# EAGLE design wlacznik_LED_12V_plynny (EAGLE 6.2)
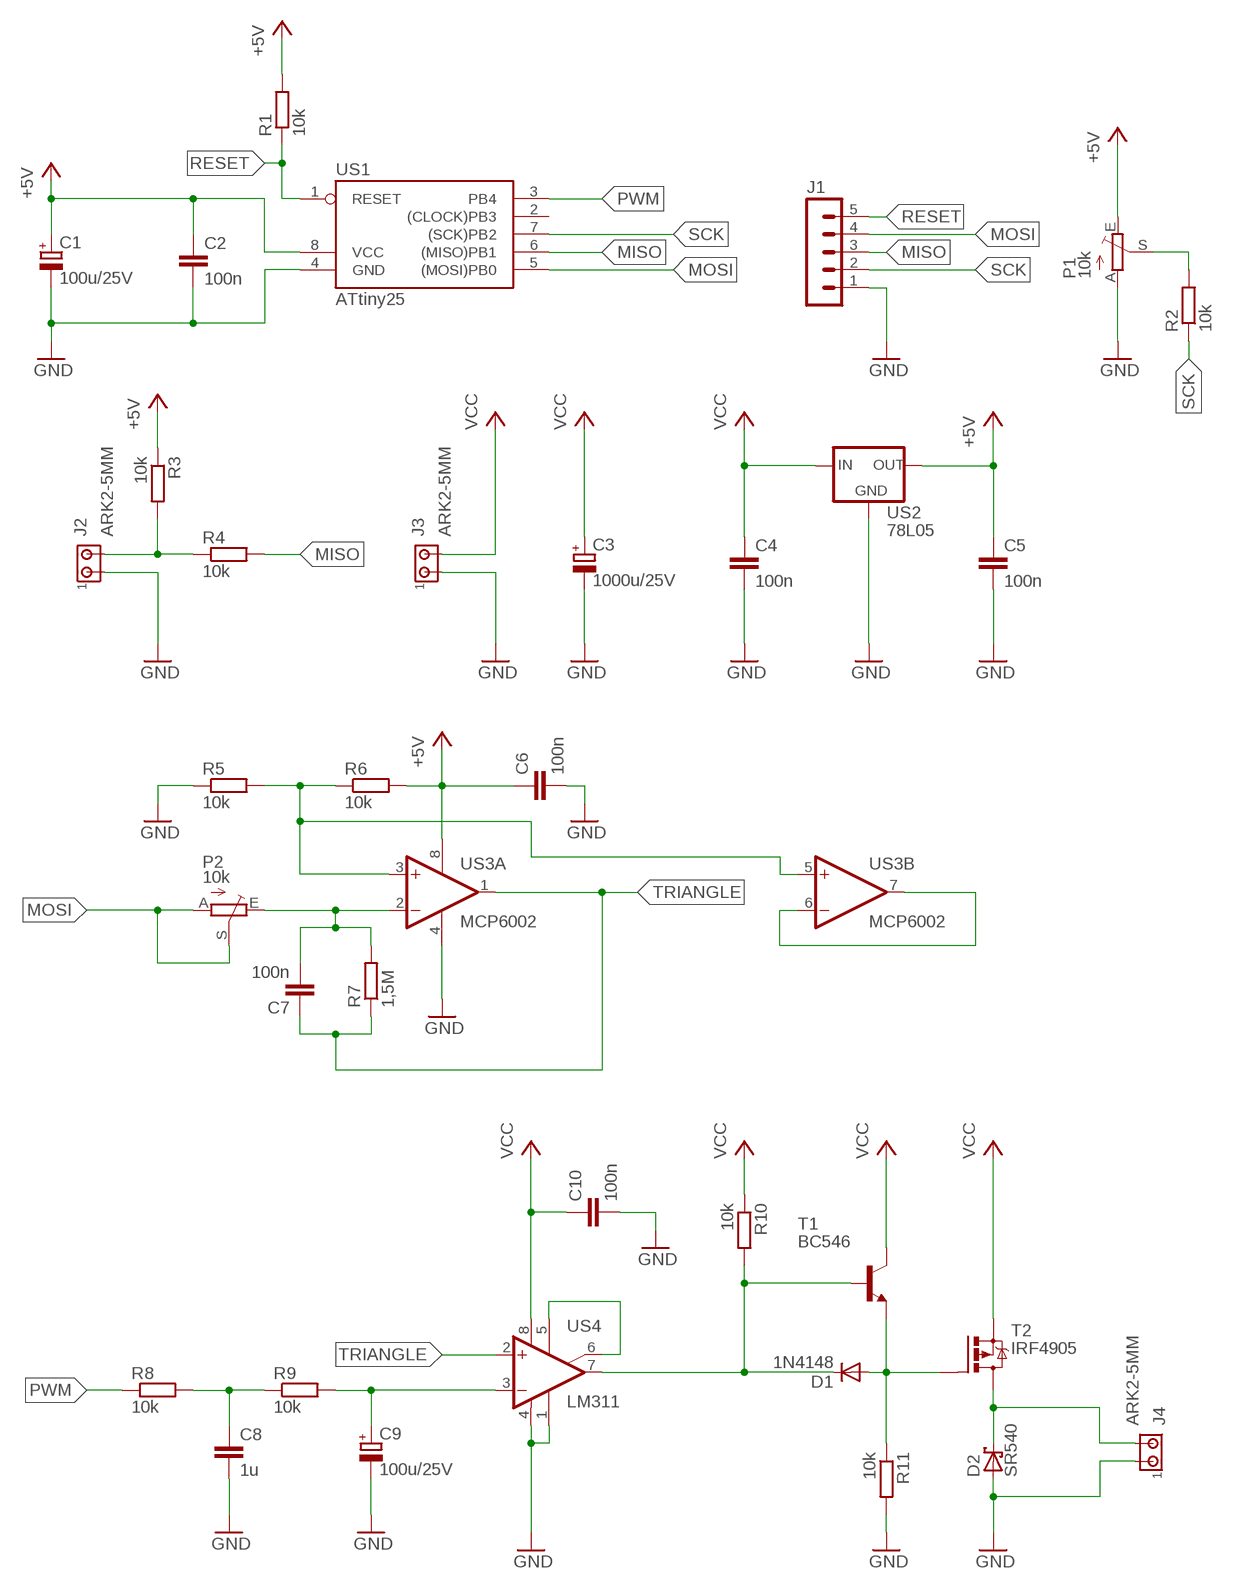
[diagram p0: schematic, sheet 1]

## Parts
C1  100u/25V  CPOL-EUE2.5-6  [E2,5-6]
C2  100n  C-EU050-025X075  [C050-025X075]
C3  1000u/25V  CPOL-EUE5-10.5  [E5-10,5]
C4  100n  C-EU050-025X075  [C050-025X075]
C5  100n  C-EU050-025X075  [C050-025X075]
C6  100n  C-EU050-025X075  [C050-025X075]
C7  100n  C-EU050-025X075  [C050-025X075]
C8  1u  C-EU050-055X075  [C050-055X075]
C9  100u/25V  CPOL-EUE2.5-6  [E2,5-6]
C10  100n  C-EU050-025X075  [C050-025X075]
D1  1N4148  1N4148DO35-7  [DO35-7]
D2  SR540  SCHOTTKY-DIODEC4111-15  [C4111-15]
J1  MA05-1  [MA05-1]
J2  ARK2-5MM  [2PIN-5MM]
J3  ARK2-5MM  [2PIN-5MM]
J4  ARK2-5MM  [2PIN-5MM]
P1  10k  TRIM_EU-CA6V  [CA6V]
P2  10k  TRIM_EU-CA6V  [CA6V]
R1  10k  R-EU_0207/7  [0207/7]
R2  10k  R-EU_0207/7  [0207/7]
R3  10k  R-EU_0207/7  [0207/7]
R4  10k  R-EU_0207/7  [0207/7]
R5  10k  R-EU_0207/7  [0207/7]
R6  10k  R-EU_0207/7  [0207/7]
R7  1,5M  R-EU_0207/7  [0207/7]
R8  10k  R-EU_0207/7  [0207/7]
R9  10k  R-EU_0207/7  [0207/7]
R10  10k  R-EU_0207/7  [0207/7]
R11  10k  R-EU_0207/7  [0207/7]
T1  BC546  BC546A  [TO92-EBC]
T2  IRF4905  IRF9530  [TO220BV]
US1  ATtiny25  TINY22P  [DIL08]
US2  78L05  78LXX  [78LXX]
US3  MCP6002  MCP602P  [DIL08]
US4  LM311  LM311N  [DIL08]

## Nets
+5V: C1.+ C2.1 C5.1 C6.1 P1.E R1.2 R3.1 R6.2 US1.8(VCC) US2.OUT US3.8(P:V+)
GND: C1.- C2.2 C3.- C4.2 C5.2 C6.2 C8.2 C9.- C10.2 D2.A J1.1 J2.P$1 J3.P$1 J4.P$1 P1.A R5.1 R11.2 US1.4(GND) US2.GND US3.4(P:V-) US4.1(GND) US4.4(V-)
MISO: J1.3 R4.2 US1.6((MISO)PB1)
MOSI: J1.4 P2.A P2.S US1.5((MOSI)PB0)
N$1: P1.S R2.2
N$2: J2.P$2 R3.2 R4.1
N$3: R5.2 R6.1 US3.3(A:+IN) US3.5(B:+IN)
N$4: D1.C R10.2 T1.B US4.7(OUT)
N$5: D1.A R11.1 T1.E T2.G
N$6: C8.1 R8.2 R9.1
N$7: D2.C J4.P$2 T2.D
N$8: C9.+ R9.2 US4.3(-IN)
N$9: US3.6(B:-IN) US3.7(B:OUT)
N$12: US4.5(ON) US4.6(ON/STR)
N$13: C7.2 P2.E R7.2 US3.2(A:-IN)
PWM: R8.1 US1.3(PB4)
RESET: J1.5 R1.1 US1.1(RESET)
SCK: J1.2 R2.1 US1.7((SCK)PB2)
TRIANGLE: C7.1 R7.1 US3.1(A:OUT) US4.2(+IN)
VCC: C3.+ C4.1 C10.1 J3.P$2 R10.1 T1.C T2.S US2.IN US4.8(V+)
Unconnected: US1.2((CLOCK)PB3)

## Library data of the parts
C1 C3 C9 = rcl:CPOL-EU: POLARIZED CAPACITOR, European symbol
C2 C4-C8 C10 = rcl:C-EU: CAPACITOR, European symbol
D1 = diode:1N4148: DIODE
D2 = diode:SCHOTTKY-DIODE: Schottky Diode
J1 = con-lstb:MA05-1: PIN HEADER; OC_FARNELL: unknown; OC_NEWARK: unknown
J2-J4 = zlacza_futrzak:ARK2: ARK 2
P1 P2 = pot:TRIM_EU-: POTENTIOMETER
R1-R11 = rcl:R-EU_: RESISTOR, European symbol
T1 = transistor-npn:BC546*: NPN Transistor
T2 = transistor-power:IRF9530: P-CHANNEL HEXFET POWER-MOS-FET Source: http://www.irf.com/product-info/datasheets/data/irf9530.pdf
US1 = atmel:TINY22: MICROCONTROLLER 1K ROM 128 bytes RAM 128 bytes EEPROM; OC_FARNELL: unknown; OC_NEWARK: unknown
US2 = v-reg:78LXX: VOLTAGE REGULATOR
US3 = linear:MCP602: Single Op Amp 2.7V to 6.0V Single Supply CMOS Source: http://ww1.microchip.com/downloads/en/DeviceDoc/21314g.pdf
US4 = linear:LM311: COMPARATOR

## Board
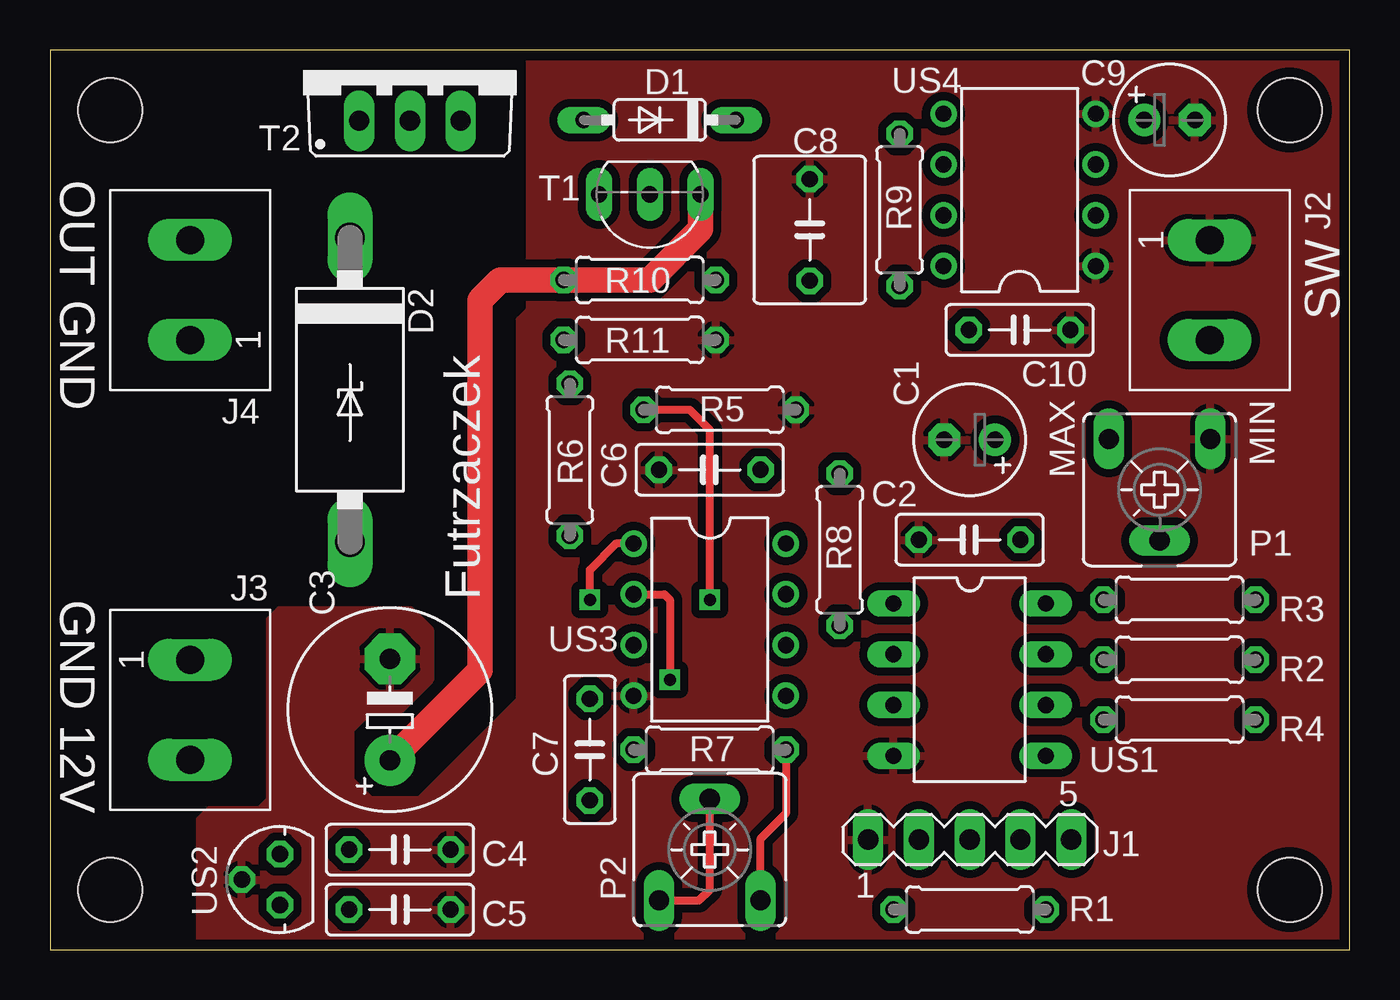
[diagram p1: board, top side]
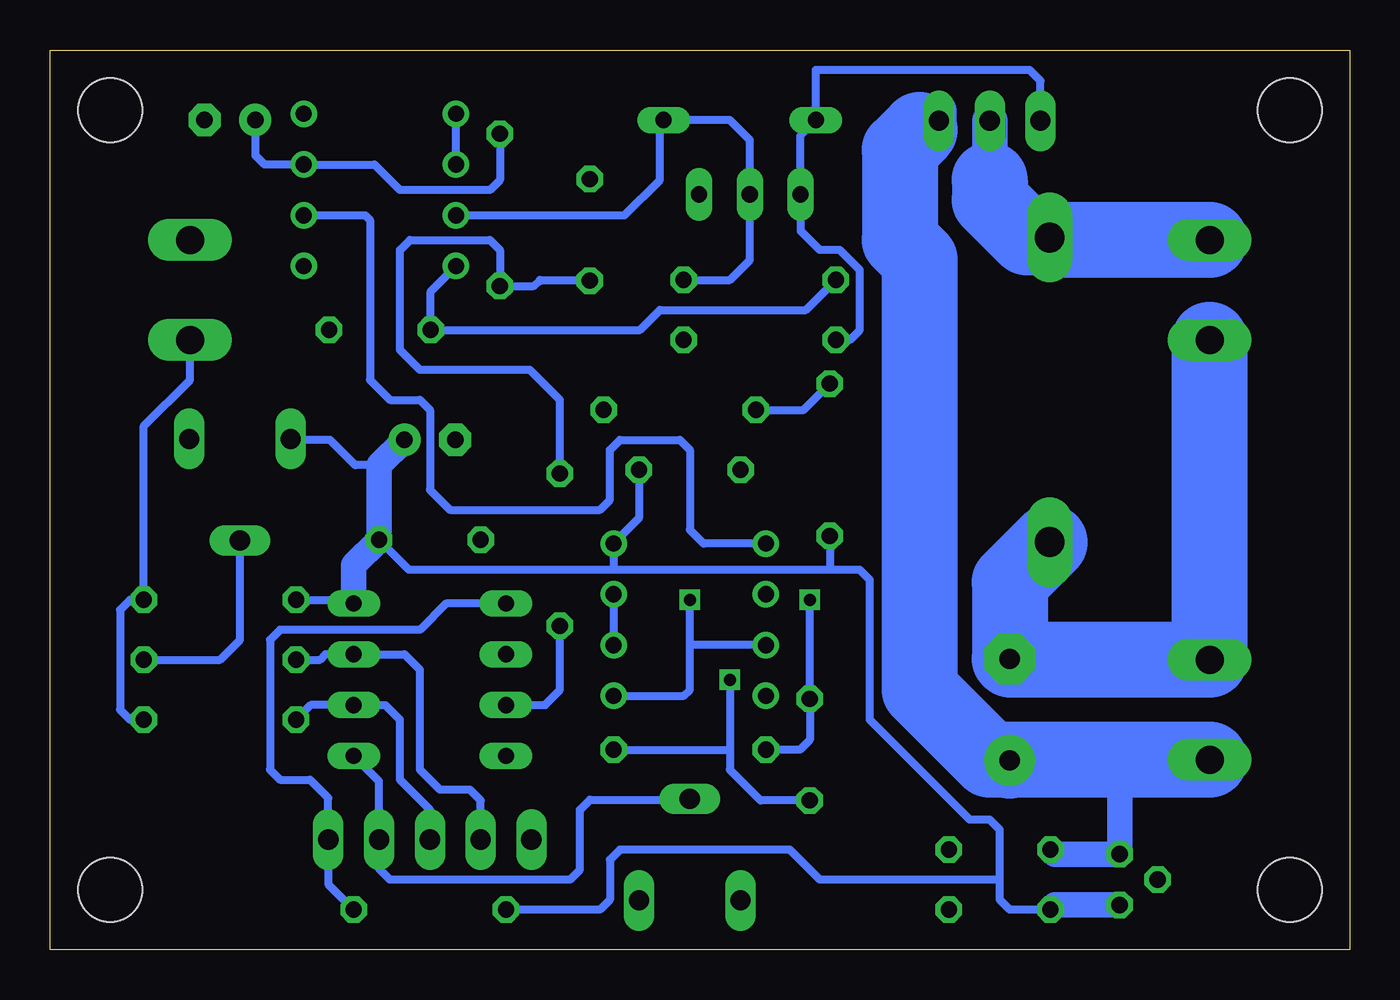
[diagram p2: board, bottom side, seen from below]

Size 65 x 45 mm. Coordinates in mm from the lower left corner, seen from the top.
Outline: 0,0 65,0 65,45 0,45 0,0
Copper layers (1*16): Top 0.035mm / dielectric 1.5mm / Bottom 0.035mm
Design rules: minimum track width 10mil, minimum drill 23mil, track to track 8mil, track to pad 8mil, pad to pad 8mil, via to via 8mil, smd to smd 8mil, copper to edge 20mil, drill to drill 8mil, minimum pad ring 10mil, minimum via ring 8mil, stop-mask expansion 4mil, vias tented up to drill 0mil, thermal gap 10mil
Holes 3.2 mm at 3,3 3,42 62,3 62,42

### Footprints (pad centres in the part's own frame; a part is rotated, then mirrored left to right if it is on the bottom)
E2,5-6 = drill 0.813 pad 1.6: + -1.27,0 | drill 0.813 pad 1.6 octagon: - 1.27,0
C050-025X075 = drill 0.813 octagon: 1 -2.54,0; 2 2.54,0
E5-10,5 = drill 1.016 pad 2.54: + -2.54,0 | drill 1.016 pad 2.54 octagon: - 2.54,0
C050-055X075 = drill 0.813 octagon: 1 -2.54,0; 2 2.54,0
DO35-7 = drill 0.813 long: A 3.81,0; C -3.81,0
C4111-15 = drill 1.499 long: A 7.62,0; C -7.62,0
MA05-1 = drill 1.016 long: 1 -5.08,0; 2 -2.54,0; 3 0,0; 4 2.54,0; 5 5.08,0
2PIN-5MM = drill 1.4 long: P$1 -2.5,0; P$2 2.5,0
CA6V = drill 1.016 long: A -2.54,-2.54; E 2.54,-2.54; S 0,2.54
0207/7 = drill 0.813 octagon: 1 -3.81,0; 2 3.81,0
TO92-EBC = drill 0.813 long: B 0,-1.27; C -2.54,-1.27; E 2.54,-1.27
TO220BV = drill 1.016 long: D 0,-2.54; G -2.54,-2.54; S 2.54,-2.54
DIL08 = drill 0.813 long: 1 -3.81,-3.81; 2 -1.27,-3.81; 3 1.27,-3.81; 4 3.81,-3.81; 5 3.81,3.81; 6 1.27,3.81; 7 -1.27,3.81; 8 -3.81,3.81
78LXX = drill 0.813 octagon: GND 0,1.905; IN 1.27,0; OUT -1.27,0
DIL08' = drill 0.813 pad 1.27: 1 -3.81,-3.81; 2 -1.27,-3.81; 3 1.27,-3.81; 4 3.81,-3.81; 5 3.81,3.81; 6 1.27,3.81; 7 -1.27,3.81; 8 -3.81,3.81

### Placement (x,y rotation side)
C1  46,25.5 180 top
C2  46,20.5 180 top
C3  17,12 90 top
C4  17.5,5 0 top
C5  17.5,2 0 top
C6  33,24 180 top
C7  27,10 270 top
C8  38,36 90 top
C9  56,41.5 0 top
C10  48.5,31 0 top
D1  30.5,41.5 180 top
D2  15,28 270 top
J1  46,5.5 0 top
J2  58,33 270 top
J3  7,12 270 top
J4  7,33 90 top
P1  55.5,23 180 top
P2  33,5 0 top
R1  46,2 180 top
R2  56.5,14.5 0 top
R3  56.5,17.5 0 top
R4  56.5,11.5 180 top
R5  33.5,27 180 top
R6  26,24.5 270 top
R7  33,10 0 top
R8  39.5,20 90 top
R9  42.5,37 90 top
R10  29.5,33.5 0 top
R11  29.5,30.5 0 top
T1  30,36.5 180 top
T2  18,44 0 top
US1  46,13.5 270 top
US2  11.5,3.5 90 top
US3  MCP6002  [DIL08']  33,16.5 270 top
US4  LM311  [DIL08']  48.5,38 90 top

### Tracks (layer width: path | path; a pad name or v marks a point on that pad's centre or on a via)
+5V
  Bottom 0.406: C5.1 17,2 17.5,2.5 17.5,3.5 | 17.5,3.5 17.5,6 18,6.5 19,6.5 24,11.5 24,18.5 24.5,19 26,19 | R3.1 50,17.5 US1.8 | 48.54,24.23 49.73,24.23 51,25.5 52.92,25.5 P1.E | 26,19 36.81,19 | 36.81,19 47.04,19 C2.1 | 17.5,3.5 26.5,3.5 28,5 36.5,5 37,4.5 37,2.5 37.5,2 R1.2 | R6.2 26,19 | 36.81,19 US3.8 35.54,21.58 C6.1
  Bottom 1.27: US2.OUT 14.73,2.23 C5.1 | US1.8 49.81,19.23 C2.1 48.54,24.23 C1.+
GND
  Bottom 3.81: J4.P$1 J3.P$1 16.96,14.5 C3.- 17,18.38 D2.A
  pour Top (isolate 0.406): 18,17 19,16 19,13.5 17.5,12 16,12 15,11 15,8.5 16,7.5 18.5,7.5 23.5,12.5 23.5,31.5 24,32 24,45 65,45 65,0 7.5,0 7.5,6.5 8,7 10.5,7 11,7.5 11,16.5 11.5,17
MISO
  Bottom 0.406: J1.3 46,7 47.5,8.5 47.5,11.5 48.23,12.23 US1.6 51.96,12.23 R4.2
MOSI
  Top 0.406: P2.A 32.46,2.46 33,3 P2.S
  Bottom 0.406: US1.5 48.54,8.42 J1.4 48.54,4.04 48,3.5 39,3.5 38.5,4 38.5,7 38,7.5 33.04,7.5 P2.S
N$1
  Bottom 0.406: R2.2 56.5,14.5 55.5,15.5 P1.S
N$2
  Bottom 0.406: R4.1 61,11.5 61.5,12 61.5,17 61,17.5 R3.2 60.31,26.19 58,28.5 J2.P$2
N$3  (via drill 0.6)
  Top 0.406: v33,17.5 33,26 32,27 R5.2
  Bottom 0.406: US3.3 33,15.23 | US3.5 33.31,12.69 33,13 33,15.23 | 33,15.23 v33,17.5 | R5.2 27.31,27 R6.1
N$4
  Bottom 0.406: T1.B 30,40.5 31,41.5 D1.C 34.5,41.31 34.5,38.5 36.27,36.73 US4.7 | 30.04,37.77 T1.B | R10.2 31,33.5 30,34.5 T1.B
N$5
  Bottom 0.406: T2.G 15.46,43.46 16,44 26.69,44 D1.A 27.46,40.73 T1.E 27.46,35.96 26.5,35 25.5,35 24.5,34 24.5,31 25,30.5 R11.1
N$6
  Bottom 0.406: R8.2 39.5,27.5 41,29 46.5,29 47.5,30 47.5,35 47,35.5 43,35.5 42.5,35 R9.1 40.81,33.19 40.5,33.5 40.46,33.46 C8.1
N$7
  Bottom 1.778: T2.D 18,38.5
  Bottom 3.81: J4.P$2 14.88,35.5 D2.C 16.12,35.62 16.5,36 18,37.5 18,38.5
N$8
  Bottom 0.406: R9.2 42.5,38.5 43,38 47.5,38 48.77,39.27 US4.3 54.27,39.27 54.73,39.73 C9.+
N$9
  Bottom 0.406: US3.7 US3.6
N$12
  Bottom 0.406: US4.6 US4.5
N$13  (via drill 0.6)
  Top 0.406: US3.2 30.73,17.77 31,17.5 v31,13.5 | P2.E 35.54,5.54 36.81,6.81 R7.2
  Bottom 0.406: v31,13.5 31,10 | 31,10 31,9 29.46,7.46 C7.2 | R7.2 31,10
PWM
  Bottom 0.406: US1.3 40.23,12.23 39.5,13 R8.1
RESET
  Bottom 0.406: R1.1 51.08,3.27 J1.5 51.08,7.58 52,8.5 53.5,8.5 54,9 54,15.5 53.5,16 46.5,16 45.19,17.31 US1.1
SCK
  Bottom 0.406: J1.2 43.46,7.46 44,8 45.5,8 46.5,9 46.5,14 47.27,14.77 US1.7 51.23,14.77 51.5,14.5 R2.1
TRIANGLE  (via drill 0.6)
  Top 0.406: v27,17.5 27,19 28.31,20.31 US3.1
  Bottom 0.406: US4.2 49.23,36.73 49,36.5 49,28.5 48,27.5 46.5,27.5 46,27 46,23 45,22 37.5,22 37,22.5 37,25 36.5,25.5 33.5,25.5 33,25 33,21 32.31,20.31 US3.1 | v27,17.5 C7.1 27,10.5 27.5,10 R7.1
VCC
  Top 1.27: C3.+ 21.5,13.96 21.5,32.5 22.5,33.5 R10.1 30,33.5 32.54,36.04 T1.C
  Bottom 0.406: US4.8 45.96,32.92 C10.1 35.5,31 34.5,32 27.19,32 R10.1
  Bottom 1.27: 12,9.5 11.5,9 US2.IN 14.73,4.77 C4.1
  Bottom 1.778: T2.S 20.54,41.96 21.5,41
  Bottom 3.81: J3.P$2 12,9.5 16.96,9.5 | 16.96,9.5 C3.+ | 16.96,9.5 18,9.5 21.5,13 21.5,34.5 22.5,35.5 22.5,40 21.5,41

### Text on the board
tPlace: OUT GND | SW | MAX | MIN | GND 12V | Futrzaczek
